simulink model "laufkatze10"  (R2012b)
settings: Solver=ode45  StartTime=0.0  StopTime=50.0  RelTol=1e-3
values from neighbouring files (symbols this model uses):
  dft = 1    [laufkatze_1.m]    (also in laufkatze_10.m = 0.1)
  F0 = 2000    [laufkatze_1.m]    (also in laufkatze_10.m)
  g = 9.89    [fuellstnd_1.m]    (also in fuellstnd_2.m; fuellstnd_21.m; fuellstnd_3.m; fuellstnd_31.m)
  JL = 400    [laufkatze_1.m]    (also in laufkatze_10.m; laufkatze_2.m; laufkatze_20.m)
  ls = 4    [laufkatze_1.m]    (also in laufkatze_10.m; laufkatze_2.m; laufkatze_20.m)
  mk = 100    [laufkatze_1.m]    (also in laufkatze_10.m; laufkatze_2.m; laufkatze_20.m)
  mL = 500    [laufkatze_1.m]    (also in laufkatze_10.m; laufkatze_2.m; laufkatze_20.m)
  mu = 0.01    [laufkatze_10.m]    (also in laufkatze_20.m; feder_masse_1.m = 0.05; feder_masse_13.m = 0.05; feder_masse_14.m = 0.05)
  Tfinal = 2000    [aktiv_tilger_1.m]    (also in aktiv_tilger_12.m = 1000; aktiv_tilger_2.m = 1000; aktiv_tilger_3.m = 1000,         dt = 0.01; aktiv_tilger_31.m = 1000,         dt = 0.01)
libraries: simulink x1

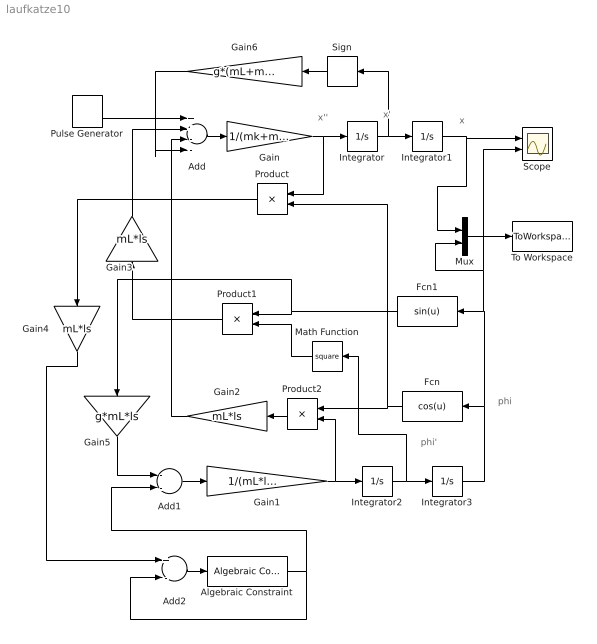
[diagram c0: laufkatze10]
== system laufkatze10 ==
  note: phi'
  note: x''
  note: x'
  note: x
  note: phi
  Add : Sum  Inputs=++--
  Add1 : Sum  Inputs=--
  Add2 : Sum  Inputs=+-
  Algebraic Constraint : simulink/Math Operations/Algebraic Constraint  z0=0
  Fcn : Fcn  Expr=cos(u)
  Fcn1 : Fcn  Expr=sin(u)
  Gain : Gain  Gain=1/(mk+mL)
  Gain1 : Gain  Gain=1/(mL*ls*ls+JL)
  Gain2 : Gain  Gain=mL*ls
  Gain3 : Gain  Gain=mL*ls
  Gain4 : Gain  Gain=mL*ls
  Gain5 : Gain  Gain=g*mL*ls
  Gain6 : Gain  Gain=g*(mL+mk)*mu
  Integrator{,1..3} (4 alike) : Integrator
  Math Function : Math  Operator=square
  Mux : Mux  Inputs=2
  Product : Product
  Product1 : Product
  Product2 : Product
  Pulse Generator : DiscretePulseGenerator  PulseType=Time based  Amplitude=F0  Period=Tfinal  PulseWidth=dft
  Scope : Scope  NumInputPorts=2
  Sign : Signum  ZeroCross=off
  To Workspace : ToWorkspace  VariableName=y  SampleTime=-1  SaveFormat=Structure With Time
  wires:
  Pulse Generator/1 -> Add/1
  Add/1 -> Gain/1
  Gain/1 -> Product/1, Integrator/1
  Integrator/1 -> Sign/1, Integrator1/1
  Add1/1 -> Gain1/1
  Gain1/1 -> Product2/2, Integrator2/1
  Integrator3/1 -> Scope/2, Mux/2, Fcn1/1, Fcn/1
  Fcn/1 -> Product/2, Product2/1
  Fcn1/1 -> Gain5/1, Product1/1
  Product2/1 -> Gain2/1
  Gain2/1 -> Add/3
  Math Function/1 -> Product1/2
  Integrator2/1 -> Math Function/1, Integrator3/1
  Product1/1 -> Gain3/1
  Gain3/1 -> Add/2
  Product/1 -> Gain4/1
  Gain5/1 -> Add1/1
  Integrator1/1 -> Mux/1, Scope/1
  Mux/1 -> To Workspace/1
  Algebraic Constraint/1 -> Add1/2, Add2/2
  Add2/1 -> Algebraic Constraint/1
  Gain4/1 -> Add2/1
  Sign/1 -> Gain6/1
  Gain6/1 -> Add/4
